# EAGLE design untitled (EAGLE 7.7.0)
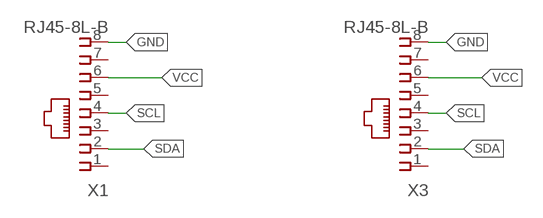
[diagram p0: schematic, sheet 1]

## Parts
X1  RJ45-8L-B  [RJ45-NO-SHIELD]
X3  RJ45-8L-B  [RJ45-NO-SHIELD]

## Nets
GND: X1.8 X3.8
SCL: X1.4 X3.4
SDA: X1.2 X3.2
VCC: X1.6 X3.6
Unconnected: X1.1 X1.3 X1.5 X1.7 X3.1 X3.3 X3.5 X3.7

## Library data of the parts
X1 X3 = con-tycoelectronics:RJ45: CORCOM Modular RJ Jacks No Shield Source: www.tycoelectronics.com .. ENG_DS_1654001_1099_RJ_L_0507.pdf; MF: TYCO ELECTRONICS; MPN: RJ45-8L-B; OC_FARNELL: 1279843; OC_NEWARK: 52K4445

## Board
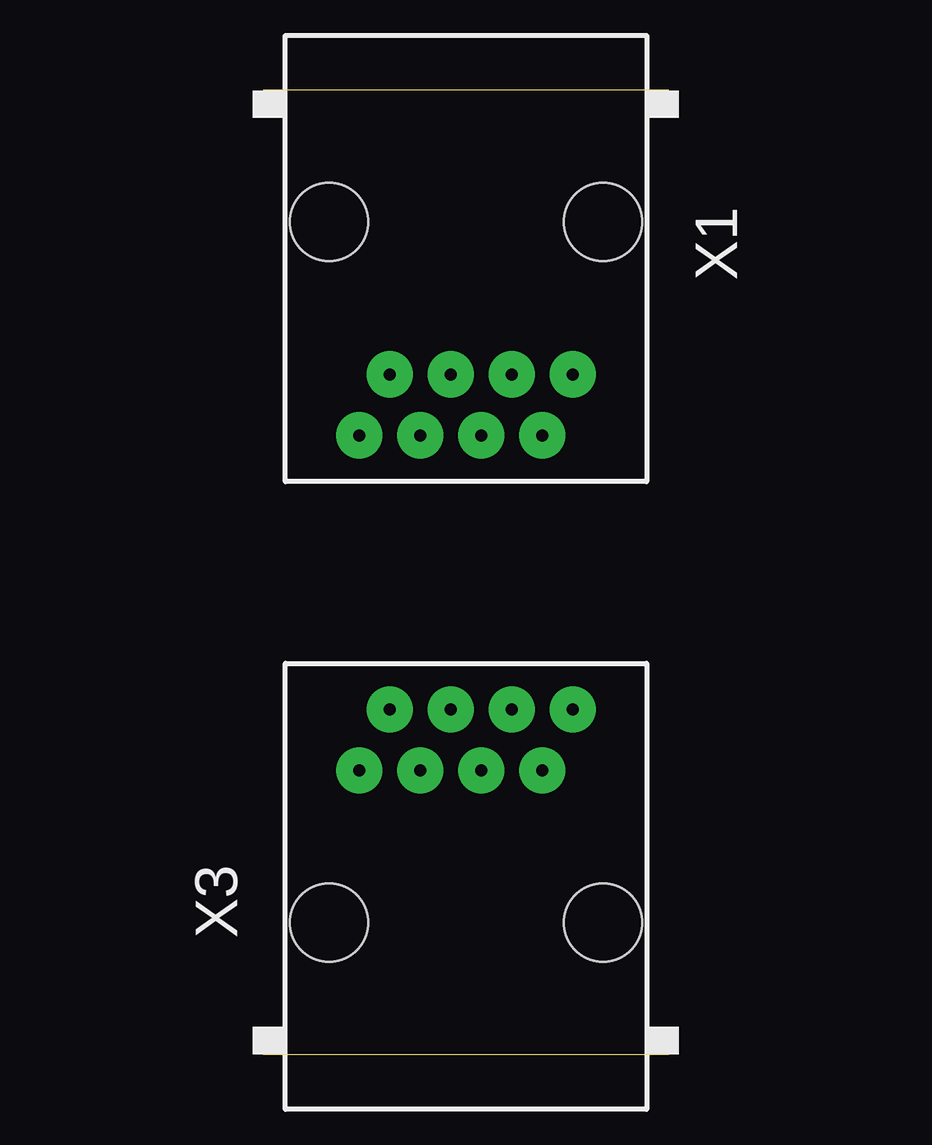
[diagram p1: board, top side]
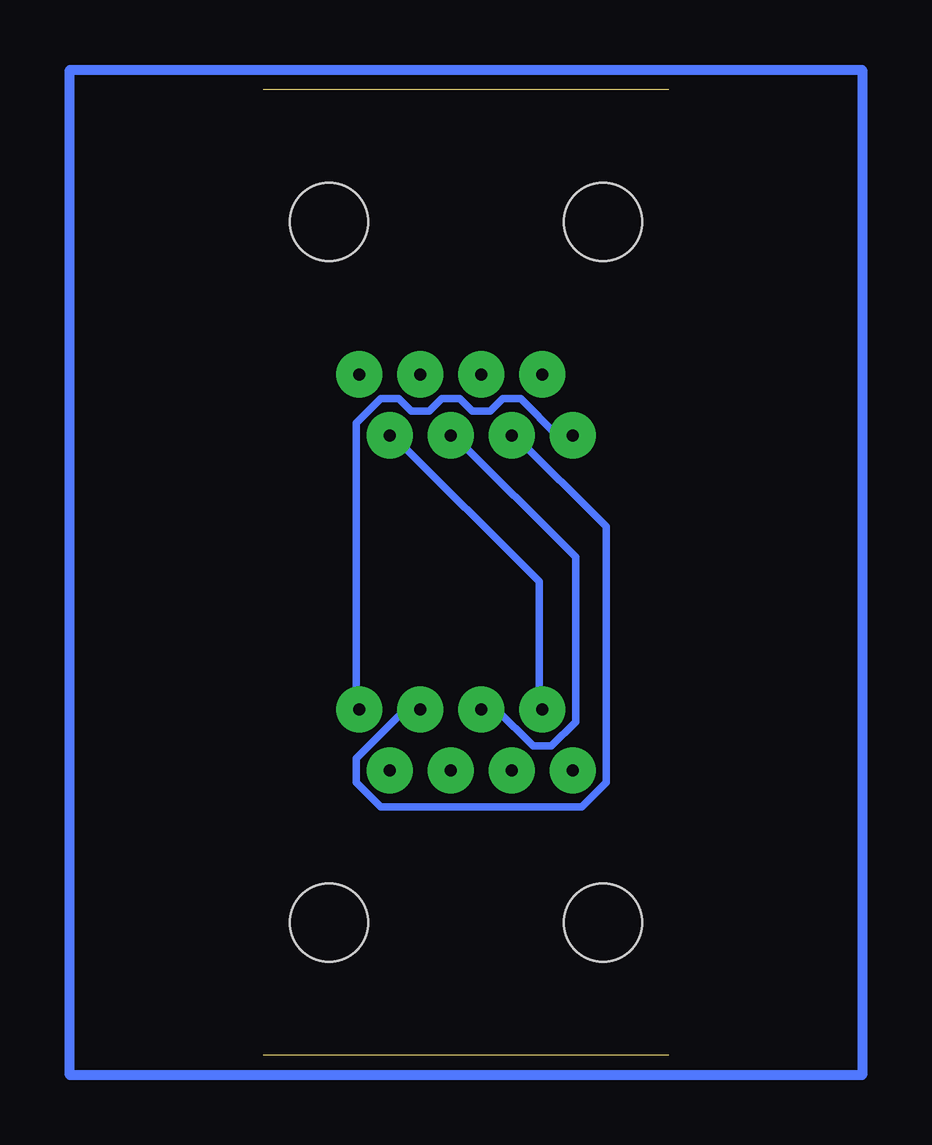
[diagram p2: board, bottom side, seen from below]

Size 16.89 x 40.23 mm. Coordinates in mm from the lower left corner, seen from the top.
Copper layers (1*16): Top 0.035mm / dielectric 1.5mm / Bottom 0.035mm
Design rules "default *": minimum track width 12mil, minimum drill 24mil, track to track 8mil, track to pad 8mil, pad to pad 8mil, via to via 8mil, smd to smd 8mil, copper to edge 40mil, drill to drill 8mil, minimum pad ring 10mil, minimum via ring 8mil, stop-mask expansion 4mil, vias tented up to drill 0mil, thermal gap 10mil

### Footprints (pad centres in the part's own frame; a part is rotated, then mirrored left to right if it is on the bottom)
RJ45-NO-SHIELD = drill 0.5 pad 1.93: 1 -4.445,6.35; 2 -3.175,8.89; 3 -1.905,6.35; 4 -0.635,8.89; 5 0.635,6.35; 6 1.905,8.89; 7 3.175,6.35; 8 4.445,8.89 | hole 3.251: -5.715,0; 5.715,0

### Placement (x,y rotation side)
X1  8.45,34.72 180 top
X3  8.45,5.51 0 top

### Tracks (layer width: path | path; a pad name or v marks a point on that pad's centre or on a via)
GND
  Bottom 0.305: X1.8 4.64,25.83 6.16,27.36 6.92,27.36 7.43,26.85 8.19,26.85 8.7,27.36 9.46,27.36 9.97,26.85 10.73,26.85 11.24,27.36 12,27.36 13.02,26.34 13.02,14.4 X3.8
N$1
  Bottom 0.406: -8.06,41.07 -8.06,-0.84 24.96,-0.84 24.96,41.07 -8.06,41.07
SCL
  Bottom 0.305: X3.4 7.18,14.4 5.65,12.88 4.89,12.88 3.87,13.89 3.87,20.75 8.95,25.83 X1.4
SDA
  Bottom 0.305: X3.2 5.4,14.4 5.4,19.74 11.49,25.83 X1.2
VCC
  Bottom 0.305: X3.6 10.99,14.4 13.02,12.37 13.02,11.35 12,10.34 3.62,10.34 2.6,11.35 2.6,22.02 6.41,25.83 X1.6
